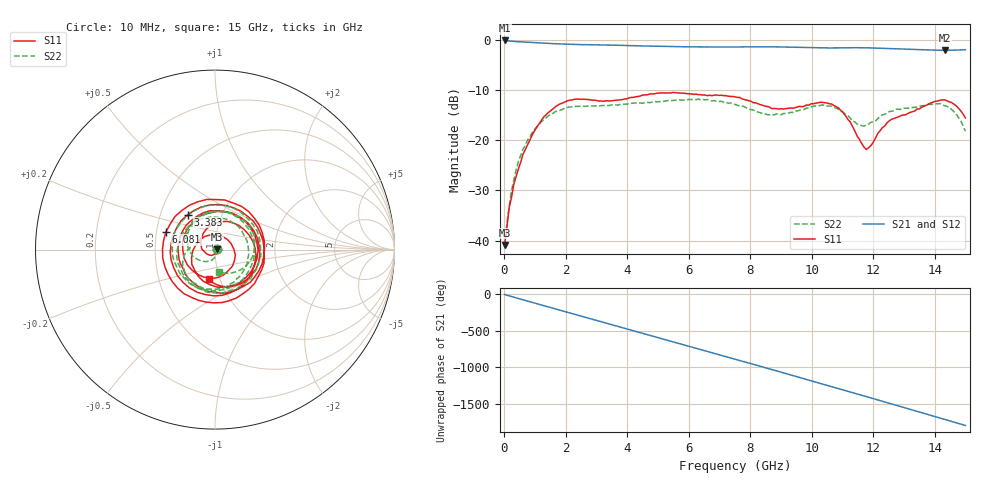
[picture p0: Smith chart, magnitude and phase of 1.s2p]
#  HZ  S  DB  R  50.00
! Rohde & Schwarz Vector Network Analyzer
! Rohde-Schwarz,ZNB3044-4Port,1351505044101548,4.21
! Created: UTC 8/5/2026, 7:46:08 PM
! freq[Hz]  db:S11  ang:S11  db:S21  ang:S21  db:S12  ang:S12  db:S22  ang:S22
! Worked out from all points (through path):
!   201 points, 10 MHz to 15 GHz, reference 50 ohm
!   highest |S21| = -0.08 dB at 10 MHz (marker M1); lowest = -2.0 dB at 14.33 GHz (marker M2)
!   group delay of S21, straight-line fit = 332 ps
!   lowest |S11| = -40.9 dB at 10 MHz (marker M3), VSWR 1.02, Z = 50.9 + j0.12 ohm
!   |S11| at or under -10 dB: start of sweep to end of sweep
!   |S22| runs from -41.1 to -11.8 dB; largest |S21 - S12| = 0.0058
!   S11 on the Smith chart (normalised r, x): 10 MHz: 1.02, +0.00; 3.383 GHz: 0.69, +0.29; 6.081 GHz: 0.56, +0.12; 15 GHz: 0.89, -0.30
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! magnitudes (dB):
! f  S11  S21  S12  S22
! 10 MHz  -40.9  -0.1  -0.1  -41.1
! 159.9 MHz  -33.4  -0.2  -0.2  -33.1
! 234.8 MHz  -31.4  -0.2  -0.2  -30.0
! 309.8 MHz  -28.7  -0.3  -0.3  -27.9
! 459.7 MHz  -25.7  -0.3  -0.3  -24.2
! 759.5 MHz  -20.9  -0.4  -0.4  -19.9
! 1.434 GHz  -14.4  -0.7  -0.7  -15.1
! 2.034 GHz  -12.2  -0.8  -0.8  -13.5
! 2.558 GHz  -11.8  -0.9  -0.9  -13.2
! 3.383 GHz  -12.1  -1.0  -1.0  -13.0
! 5.032 GHz  -10.6  -1.2  -1.2  -12.3
! 6.081 GHz  -10.7  -1.3  -1.3  -11.9
! 7.505 GHz  -11.3  -1.4  -1.4  -12.8
! 8.629 GHz  -13.4  -1.3  -1.3  -14.9
! 10.05 GHz  -12.7  -1.5  -1.5  -13.2
! 10.88 GHz  -13.6  -1.6  -1.5  -13.8
! 11.48 GHz  -19.1  -1.5  -1.5  -16.7
! 11.78 GHz  -21.8  -1.5  -1.5  -16.9
! 12.53 GHz  -16.1  -1.7  -1.7  -14.2
! 14.33 GHz  -11.9  -2.0  -2.0  -13.1
! 14.7 GHz  -13.1  -2.0  -2.0  -14.8
! 15 GHz  -15.5  -1.9  -1.9  -18.2
